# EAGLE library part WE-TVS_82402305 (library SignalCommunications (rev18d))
TVS Diode Standard Series Characteristics Operating temperature: –55 ºC to +85 °C for 824 023 x; –55 ºC to +125 °C for 824 021/824 022 Very low clamping voltage High ESD withstand voltage Unidirectional or bidirectional protection RoHS, REACH and free of halogens Applications DC power supply Headsets and accessories PDAs Digital cameras MP3-Player Touch Panels ESD protection in accordance with EN 61000-4-2 – 8 kV contact discharge – 15 kV air discharge Details see: http://katalog.we-online.de/en/pbs/WE-TVS_High_Speed/824021? Updated by Dan Xu 2014-07-11 2014 (C) Wurth Elektronik
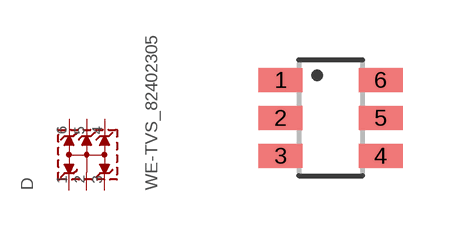
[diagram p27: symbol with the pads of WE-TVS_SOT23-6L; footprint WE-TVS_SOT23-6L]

Designator prefix D

## WE-TVS_82402305  [WE-TVS_SOT23-6L]
1  1  pas
2  GND  pas
3  2  pas
4  3  pas
5  4  pas
6  5  pas

## Footprint WE-TVS_SOT23-6L (pad centres in mm)
TVS Diode Array WE-TVS
smd 1.1 x 0.6: 1 -1.25,0.95; 2 -1.25,0; 3 -1.25,-0.95; 4 1.25,-0.95; 5 1.25,0; 6 1.25,0.95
